FUNCTION FC 70 : VOID
TITLE =Program management
VERSION : 0.1

BEGIN
NETWORK
TITLE =Start loading of program
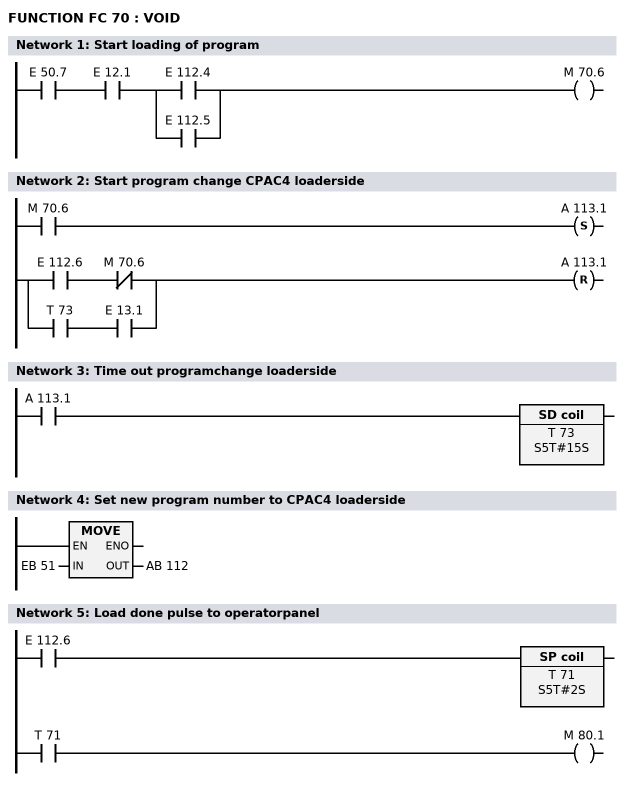
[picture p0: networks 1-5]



//      U(
      U     E     50.7;
//      BLD   100
//      FP    "M70.5"
//      )
      U     E     12.1;
      U(    ;
      O     E    112.4;
      O     E    112.5;
      )     ;
      =     M     70.6;
NETWORK
TITLE =Start program change CPAC4 loaderside

      U     M     70.6;
      S     A    113.1;
      U(    ;
      U     E    112.6;
      UN    M     70.6;
      O     ;
      U     T     73;
      U     E     13.1;
      )     ;
      R     A    113.1;
      NOP   0;
NETWORK
TITLE =Time out programchange loaderside

      U     A    113.1;
      L     S5T#15S;
      SE    T     73;
      NOP   0;
      NOP   0;
      NOP   0;
      NOP   0;
NETWORK
TITLE =Set new program number to CPAC4 loaderside

      L     EB    51;
      T     AB   112;
      NOP   0;
NETWORK
TITLE =Load done pulse to operatorpanel

      U     E    112.6;
      L     S5T#2S;
      SI    T     71;
      NOP   0;
      NOP   0;
      NOP   0;
      U     T     71;
      =     M     80.1;
END_FUNCTION

